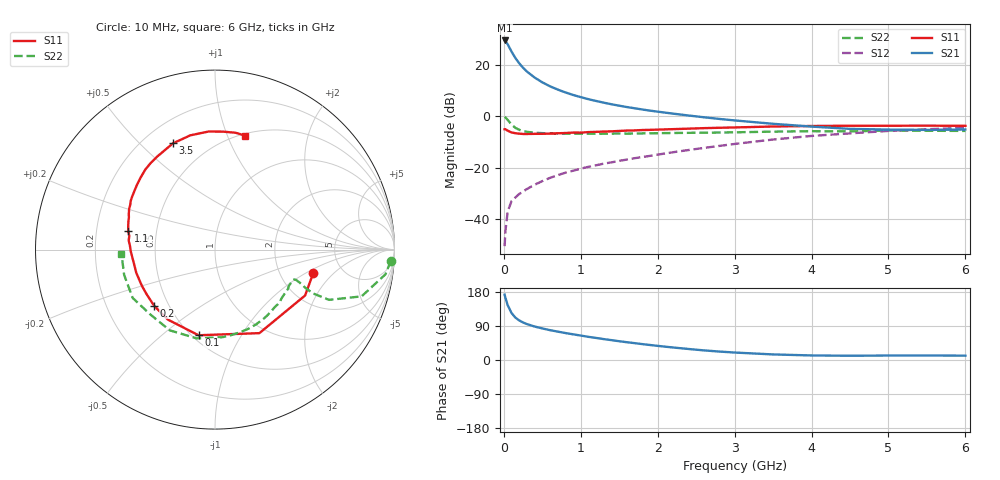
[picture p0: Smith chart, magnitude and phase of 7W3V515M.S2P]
! Infineon Technologies  Discrete & RF Semiconductors
! BFS17W
! Si NPN RF Bipolar Junction Transistor in SOT323
! VCE = 3.5 V  IC = 15 mA
! Common Emitter S-Parameters:  August  1999
# GHz  S  MA  R  50
!  f  S11  S21  S12  S22
! GHz  MAG  ANG  MAG  ANG  MAG  ANG  MAG  ANG
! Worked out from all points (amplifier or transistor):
!   36 points, 10 MHz to 6 GHz, reference 50 ohm
!   highest |S21| = 29.7 dB at 10 MHz (marker M1)
!   |S21| within 3 dB of that: start of sweep to 76.28 MHz
!   unconditionally stable (mu >= 1): 325.5 MHz to 2.352 GHz; 4.747 GHz to end of sweep
!   at 250 MHz: K = 0.91, MSG = 24.2 dB, |S12| = -29.4 dB
!   at 1.4 GHz: K = 1.20, MAG = 8.7 dB, |S12| = -18.0 dB
!   at 6 GHz: K = 1.06, MAG = -1.9 dB, |S12| = -4.4 dB
!   S11 on the Smith chart (normalised r, x): 10 MHz: 3.07, -1.18; 100 MHz: 0.54, -0.67; 200 MHz: 0.42, -0.33; 1.1 GHz: 0.34, +0.10; 3.5 GHz: 0.32, +0.63; 6 GHz: 0.52, +1.16
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0.01  0.5628 -13.5  30.72 172.4  0.0029 77.8  0.9815 -3.7
0.02  0.5633 -27.0  29.98 164.4  0.0056 82.7  0.9592 -8.3
0.05  0.5271 -62.0  25.84 144.6  0.0138 66.9  0.8572 -17.7
0.1  0.486 -100.9  18.61 123.9  0.0221 58.6  0.6939 -23.8
0.15  0.4703 -124.0  13.91 111.9  0.026 55.1  0.5992 -24.1
0.2  0.4613 -137.5  10.98 104.4  0.0305 57.2  0.5489 -23.0
0.25  0.4549 -146.9  8.976 99.0  0.0338 57.9  0.518 -21.8
0.3  0.4545 -153.7  7.582 94.8  0.0381 60.6  0.5015 -21.1
0.4  0.4574 -163.6  5.781 88.3  0.0461 62.6  0.4801 -20.5
0.5  0.458 -169.8  4.659 83.3  0.0544 65.2  0.4722 -20.6
0.6  0.4628 -174.7  3.894 78.8  0.0629 66.3  0.4664 -21.5
0.7  0.4694 -178.9  3.364 74.9  0.0711 67.4  0.4626 -22.9
0.9  0.4836 174.0  2.638 67.8  0.0868 68.5  0.4586 -26.4
1.1  0.4947 167.7  2.18 61.1  0.1037 68.6  0.4598 -30.8
1.3  0.5074 161.9  1.862 55.1  0.1197 69.4  0.4591 -35.7
1.6  0.53 154.4  1.528 46.9  0.1436 69.7  0.4622 -43.5
2.2  0.5651 140.3  1.136 33.0  0.1996 70.0  0.475 -60.9
2.8  0.6011 126.5  0.896 22.3  0.2654 67.5  0.485 -79.4
3.5  0.6367 111.6  0.719 14.7  0.3541 61.7  0.505 -101.7
4.5  0.6588 93.2  0.572 11.2  0.467 49.0  0.5105 -135.2
5.5  0.6611 80.0  0.546 11.9  0.5626 36.2  0.5254 -164.5
6  0.6565 75.0  0.556 11.5  0.6004 30.1  0.5216 -177.3
